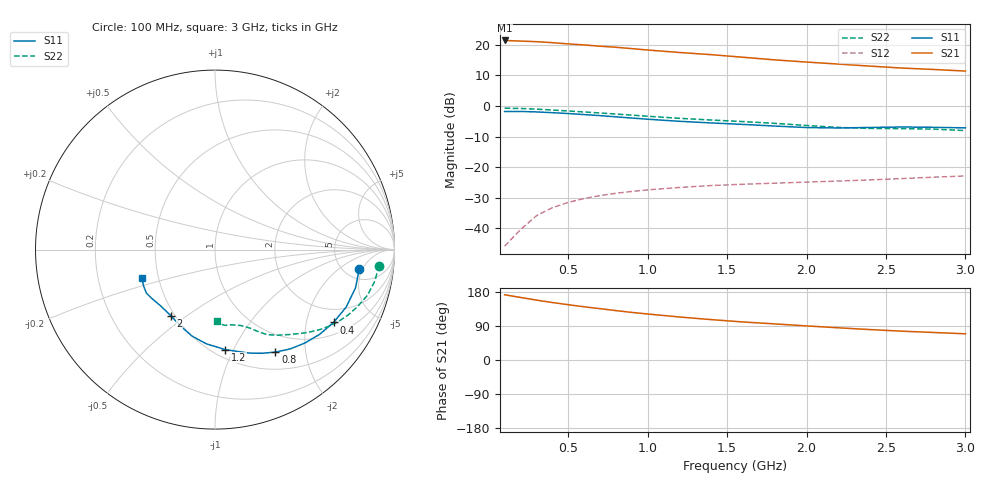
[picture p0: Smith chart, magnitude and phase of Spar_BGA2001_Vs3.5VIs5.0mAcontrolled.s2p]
! Filename: 35G1.001
! Title: BGA2001 X0297-20 HFE=80
! Bias: Vce=3V; Ic=5.0mA controlled / noise data included
! Company: NXP Semiconductors NL
! User: Quality&Reliability T&D
! Measure time: 23 Oct 1998 / 08:34:00
#  MHz  S  MA  R 50
! Freq  S11  S21  S12  S22  :
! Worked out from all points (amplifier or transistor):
!   20 points, 100 MHz to 3 GHz, reference 50 ohm
!   highest |S21| = 21.4 dB at 100 MHz (marker M1)
!   |S21| within 3 dB of that: start of sweep to 973.2 MHz
!   unconditionally stable (mu >= 1): 1.988 GHz to end of sweep
!   at 400 MHz: K = 0.24, MSG = 27.0 dB, |S12| = -33.3 dB
!   at 1.2 GHz: K = 0.59, MSG = 22.1 dB, |S12| = -26.7 dB
!   at 3 GHz: K = 1.24, MAG = 14.2 dB, |S12| = -22.9 dB
!   lowest NFmin = 1.30 dB at 1.8 GHz
!   S11 on the Smith chart (normalised r, x): 100 MHz: 6.90, -4.26; 400 MHz: 1.42, -2.90; 800 MHz: 0.73, -1.49; 1.2 GHz: 0.57, -0.93; 2 GHz: 0.48, -0.44; 3 GHz: 0.40, -0.16
100  0.8108 -7.5  11.74 172.1  0.005104 59.2  0.917 -5.6
200  0.8115 -15.2  11.47 165.0  0.009497 78.4  0.9082 -11.1
300  0.798 -23.6  11.21 158.1  0.01605 78.3  0.8867 -16.7
400  0.7752 -31.6  10.81 151.7  0.02167 74.0  0.8561 -21.7
500  0.7503 -39.0  10.32 145.9  0.02651 69.9  0.8265 -26.2
600  0.7222 -46.1  9.921 140.5  0.03061 66.4  0.796 -30.2
700  0.6945 -52.8  9.461 135.4  0.03422 63.5  0.7664 -33.8
800  0.663 -59.5  9.09 130.4  0.03736 60.9  0.7365 -37.1
900  0.6337 -65.7  8.634 125.6  0.03998 58.7  0.707 -40.2
1000  0.6063 -71.9  8.199 121.4  0.04248 57.0  0.6785 -43.3
1200  0.5606 -84.0  7.467 113.5  0.04647 54.1  0.6272 -49.0
1400  0.5269 -95.3  6.883 106.6  0.04997 52.1  0.5883 -54.2
1600  0.4987 -104.8  6.244 100.4  0.05249 51.5  0.5547 -58.5
1800  0.4686 -113.8  5.654 95.2  0.05464 52.0  0.519 -62.0
2000  0.4429 -123.8  5.208 90.0  0.05688 51.9  0.4786 -66.0
2200  0.436 -134.1  4.826 85.0  0.05921 51.7  0.4452 -71.6
2400  0.4447 -142.1  4.472 80.3  0.06177 52.5  0.4287 -77.8
2600  0.4527 -147.6  4.157 76.1  0.06487 54.1  0.4259 -82.4
2800  0.447 -152.6  3.941 72.6  0.06844 54.7  0.4176 -85.2
3000  0.4378 -158.7  3.712 69.1  0.07173 55.6  0.3953 -88.0
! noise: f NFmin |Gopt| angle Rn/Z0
900  1.34  0.33  20.6  0.28
1000  1.36  0.31  20.5  0.3
1800  1.299  0.279  66.18  0.234
2000  1.331  0.27  72.85  0.234
2200  1.442  0.222  84.7  0.231
2400  1.557  0.207  101.7  0.209
